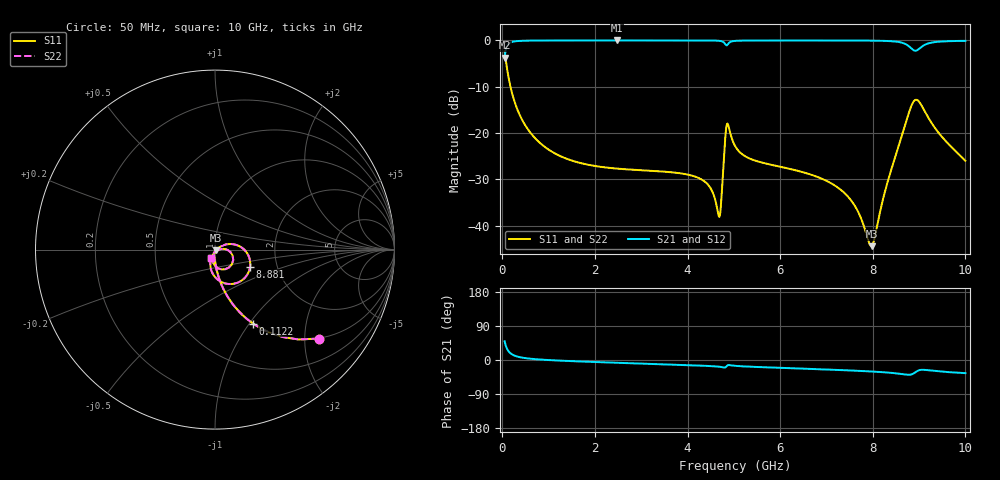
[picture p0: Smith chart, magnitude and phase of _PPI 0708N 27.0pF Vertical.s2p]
! S-Parameter data specifications (vertical orientation):
! Substrate: 40-mil Rogers 3003C, Substrate thickness, H=1.016mm, Dielectric constant, Er=3, Conductor thickness, T_mtl=0.043mm, Loss Tangent, Tand=0.003
! PCB Mounting Pad Footprint: Pad width, PadW=2.54mm , Pad length, PadL=0.51mm , Pad gap, PadG (edge-to-edge)=0.71mm , Reference planes=1.73mm apart
! Created Tue Jan 16 08:52:53 2018
# GHz S MA R 50
! 2 Port Network Data from SP1.SP block
! freq  magS11  angS11  magS21  angS21  magS12  angS12  magS22  angS22
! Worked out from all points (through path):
!   801 points, 50 MHz to 10 GHz, reference 50 ohm
!   highest |S21| = -0.01 dB at 2.475 GHz (marker M1); lowest = -3.8 dB at 50 MHz (marker M2)
!   group delay of S21, straight-line fit = 11.9 ps
!   lowest |S11| = -44.4 dB at 7.973 GHz (marker M3), VSWR 1.01, Z = 50.5 - j0.388 ohm
!   |S11| at or under -10 dB: 176.5 MHz to end of sweep
!   |S22| runs from -44.4 to -2.4 dB; largest |S21 - S12| = 0
!   S11 on the Smith chart (normalised r, x): 50 MHz: 0.99, -2.33; 112.2 MHz: 0.99, -1.04; 8.881 GHz: 1.45, -0.30; 10 GHz: 0.96, -0.09
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0.05  0.7607 -40.7  0.649 49.3  0.649 49.3  0.7607 -40.7
0.1121875  0.4634 -62.8  0.8859 27.2  0.8859 27.2  0.4634 -62.8
0.3111875  0.1873 -80.4  0.9821 9.6  0.9821 9.6  0.1873 -80.4
0.622125  0.09855 -86.6  0.9948 3.2  0.9948 3.2  0.09855 -86.6
1.716625  0.04701 -93.5  0.9984 -4.0  0.9984 -4.0  0.04701 -93.5
2.475312  0.04128 -96.6  0.9985 -7.3  0.9985 -7.3  0.04128 -96.6
3.370812  0.03866 -100.0  0.9985 -10.9  0.9985 -10.9  0.03866 -100.0
4.3285  0.03095 -102.2  0.9978 -15.1  0.9978 -15.1  0.03095 -102.2
4.67675  0.0126 -58.3  0.9902 -17.7  0.9902 -17.7  0.0126 -58.3
4.7265  0.01799 -8.9  0.9821 -18.5  0.9821 -18.5  0.01799 -8.9
4.801125  0.071 -1.9  0.932 -19.9  0.932 -19.9  0.071 -1.9
4.850875  0.1251 -41.8  0.886 -15.7  0.886 -15.7  0.1251 -41.8
5.025  0.07272 -97.9  0.9877 -15.3  0.9877 -15.3  0.07272 -97.9
5.398125  0.05163 -105.6  0.9964 -17.9  0.9964 -17.9  0.05163 -105.6
6.691625  0.03518 -111.0  0.9975 -23.7  0.9975 -23.7  0.03518 -111.0
7.487625  0.01995 -109.2  0.9966 -27.5  0.9966 -27.5  0.01995 -109.2
7.972688  0.005999 -39.9  0.9938 -30.3  0.9938 -30.3  0.005999 -39.9
8.345812  0.03275 28.7  0.9839 -33.3  0.9839 -33.3  0.03275 28.7
8.7065  0.1261 11.1  0.9132 -38.5  0.9132 -38.5  0.1261 11.1
8.880625  0.2183 -26.4  0.7835 -35.6  0.7835 -35.6  0.2183 -26.4
9.216437  0.1418 -93.3  0.9335 -27.3  0.9335 -27.3  0.1418 -93.3
10  0.05009 -113.9  0.989 -34.7  0.989 -34.7  0.05009 -113.9
